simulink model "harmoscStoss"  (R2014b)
settings: Solver=ode45  StartTime=0.0  StopTime=20.0  RelTol=1e-3
PreLoadFcn:
  | disp('omega=1 in PreLoadFcn gesetzt')
  | omega=1;

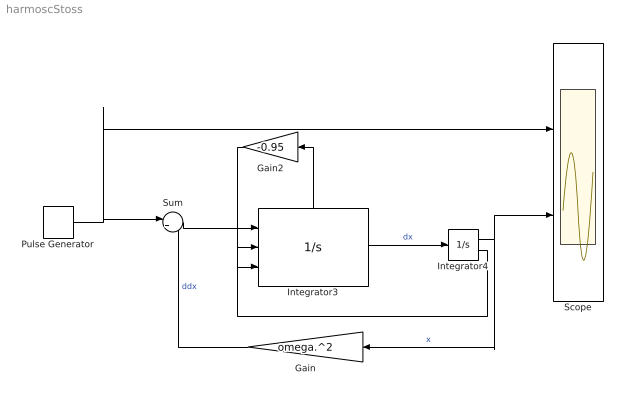
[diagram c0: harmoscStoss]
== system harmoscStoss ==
  Gain : Gain  Gain=omega.^2
  Gain2 : Gain  Gain=-0.95
  Integrator3 : Integrator  ExternalReset=either  InitialConditionSource=external  ShowStatePort=on
  Integrator4 : Integrator  LimitOutput=on  UpperSaturationLimit=[0.25, inf]  ShowSaturationPort=on
  Pulse Generator : DiscretePulseGenerator  PulseType=Time based  Period=2*pi/omega  PulseWidth=5
  Scope : Scope  NumInputPorts=2
  Sum : Sum  Inputs=|+-
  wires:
  Integrator3/1 -> Integrator4/1  "dx"
  Integrator4/1 -> Scope/2, Gain/1  "x"
  Sum/1 -> Integrator3/1
  Pulse Generator/1 -> Scope/1, Sum/1
  Gain/1 -> Sum/2  "ddx"
  Integrator4/2 -> Integrator3/2
  Gain2/1 -> Integrator3/3
  Integrator3/State -> Gain2/1
